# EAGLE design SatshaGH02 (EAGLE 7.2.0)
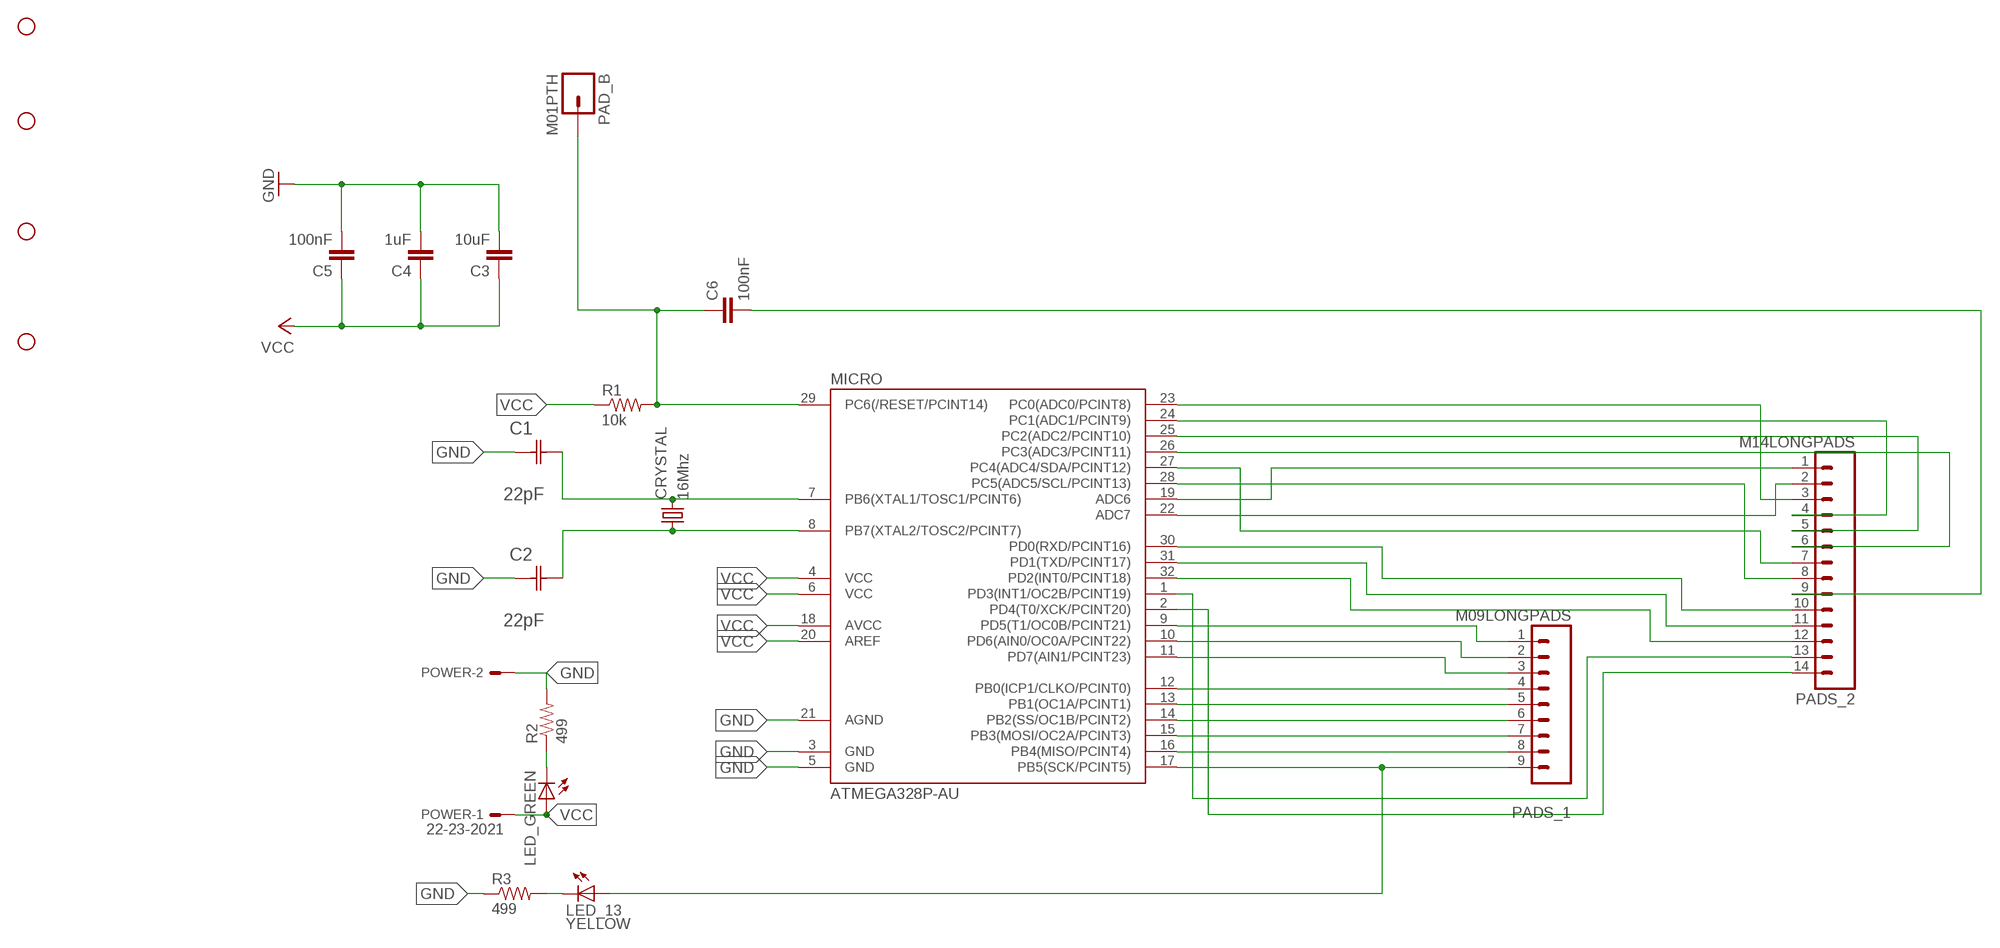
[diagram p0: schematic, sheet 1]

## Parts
C1  22pF  0612ZC225MAT2A  [CAPC3216X178N]
C2  22pF  0612ZC225MAT2A  [CAPC3216X178N]
C3  10uF  CAP1206  [1206]
C4  1uF  CAP1206  [1206]
C5  100nF  CAP1206  [1206]
C6  100nF  CAP1206  [1206]
CRYSTAL  16Mhz  CSM-7X-DU  [CSM-7X-DU]
LED_13  YELLOW  LED1206  [1206]
LED_GREEN  LED1206  [1206]
MICRO  ATMEGA328P-AU  ATMEGA48/88/168-AU  [TQFP32-08]
PAD_B  M01PTH  [1X01]
PADS_1  M09LONGPADS  [1X09_LONGPADS]
PADS_2  M14LONGPADS  [1X14-LONGPADS]
POWER  22-23-2021  [22-23-2021]
R1  10k  RESISTOR1206  [1206]
R2  499  RESISTOR1206  [1206]
R3  499  RESISTOR1206  [1206]
U$1  STAND-OFF  [STAND-OFF]
U$2  STAND-OFF  [STAND-OFF]
U$3  STAND-OFF  [STAND-OFF]
U$4  STAND-OFF  [STAND-OFF]

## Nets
GND: C1.1(C1) C2.1(C1) C3.2 C4.2 C5.2 MICRO.3(GND) MICRO.5(GND) MICRO.21(AGND) POWER.2 R2.2 R3.1
N$1: MICRO.9(PD5(T1/OC0B/PCINT21)) PADS_1.1
N$2: C1.2(C2) CRYSTAL.2 MICRO.7(PB6(XTAL1/TOSC1/PCINT6))
N$3: C6.2 PADS_2.9
N$4: MICRO.10(PD6(AIN0/OC0A/PCINT22)) PADS_1.2
N$5: MICRO.11(PD7(AIN1/PCINT23)) PADS_1.3
N$6: MICRO.12(PB0(ICP1/CLKO/PCINT0)) PADS_1.4
N$7: MICRO.13(PB1(OC1A/PCINT1)) PADS_1.5
N$8: MICRO.14(PB2(SS/OC1B/PCINT2)) PADS_1.6
N$9: C2.2(C2) CRYSTAL.1 MICRO.8(PB7(XTAL2/TOSC2/PCINT7))
N$10: MICRO.15(PB3(MOSI/OC2A/PCINT3)) PADS_1.7
N$11: MICRO.16(PB4(MISO/PCINT4)) PADS_1.8
N$12: LED_13.1(A) MICRO.17(PB5(SCK/PCINT5)) PADS_1.9
N$13: MICRO.19(ADC6) PADS_2.1
N$14: MICRO.22(ADC7) PADS_2.2
N$15: MICRO.23(PC0(ADC0/PCINT8)) PADS_2.3
N$16: MICRO.24(PC1(ADC1/PCINT9)) PADS_2.4
N$17: MICRO.25(PC2(ADC2/PCINT10)) PADS_2.5
N$18: MICRO.26(PC3(ADC3/PCINT11)) PADS_2.6
N$19: MICRO.27(PC4(ADC4/SDA/PCINT12)) PADS_2.7
N$20: MICRO.30(PD0(RXD/PCINT16)) PADS_2.10
N$21: MICRO.31(PD1(TXD/PCINT17)) PADS_2.11
N$22: MICRO.32(PD2(INT0/PCINT18)) PADS_2.12
N$23: MICRO.1(PD3(INT1/OC2B/PCINT19)) PADS_2.13
N$24: MICRO.2(PD4(T0/XCK/PCINT20)) PADS_2.14
N$25: MICRO.28(PC5(ADC5/SCL/PCINT13)) PADS_2.8
N$26: LED_GREEN.2(C) R2.1
N$27: LED_13.2(C) R3.2
N$28: C6.1 MICRO.29(PC6(/RESET/PCINT14)) PAD_B.1 R1.2
VCC: C3.1 C4.1 C5.1 LED_GREEN.1(A) MICRO.4(VCC) MICRO.6(VCC) MICRO.18(AVCC) MICRO.20(AREF) POWER.1 R1.1

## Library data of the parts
C1 C2 = AVX_By_element14_Batch_1:0612ZC225MAT2A: Capacitor 1206; MPN: 0612ZC225MAT2A; OC_FARNELL: -; OC_NEWARK: 12N3209; SUPPLIER: AVX; TOLERANCE: ±20%; VALUE: 2.2µF; VOLTAGERATING: 10V
C3-C6 = 01_SparkFun:CAP: Capacitor
CRYSTAL = 01_FAB_Hello:CSM-7X-DU: SMD CRYSTAL; OC_FARNELL: unknown; OC_NEWARK: unknown
LED_13 LED_GREEN = 01_FAB_Hello:LED
MICRO = atmega8:ATMEGA48/88/168
PAD_B = 01_SparkFun:M01: Header 1
PADS_1 = 01_SparkFun:M09: Header 9 Standard 9-pin 0.1" header. Use with straight break away headers (SKU : PRT-00116), right angle break away headers (PRT-00553), swiss pins (PRT-00743), machine pins (PRT-00117), and female headers (PRT-00115).
PADS_2 = 01_SparkFun:M14: Header 14 Standard 14-pin 0.1" header. Use with straight break away headers (SKU : PRT-00116), right angle break away headers (PRT-00553), swiss pins (PRT-00743), machine pins (PRT-00117), and female headers (PRT-00115).
POWER = con-molex:22-23-2021: .100" (2.54mm) Center Header - 2 Pin; MF: MOLEX; MPN: 22-23-2021; OC_FARNELL: 1462926; OC_NEWARK: 25C3832
R1-R3 = 01_SparkFun:RESISTOR: Resistor
U$1-U$4 = SparkFun:STAND-OFF: Stand Off

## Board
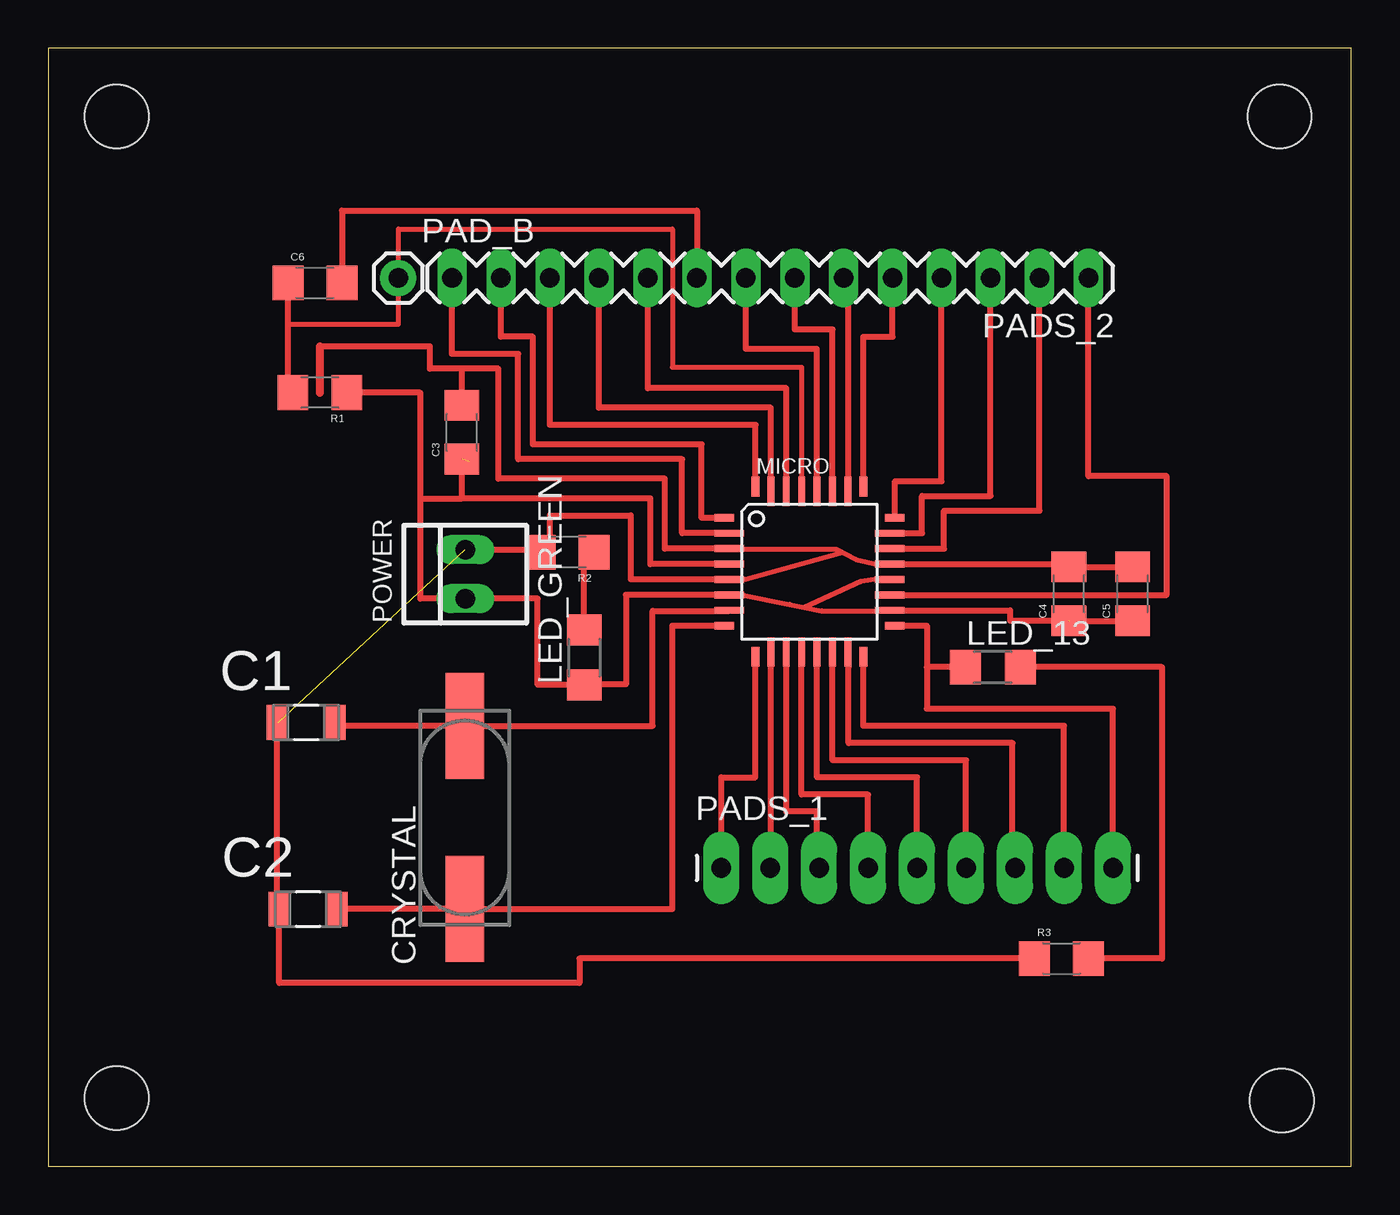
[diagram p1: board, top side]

Size 67.62 x 58.03 mm. Coordinates in mm from the lower left corner, seen from the top.
Outline: 0,0 67.62,0 67.62,58.03 0,58.03 0,0
Copper layers (1*16): Top 0.035mm / dielectric 1.5mm / Bottom 0.035mm
Design rules "default": minimum track width 10mil, minimum drill 24mil, track to track 8mil, track to pad 8mil, pad to pad 8mil, via to via 8mil, smd to smd 8mil, copper to edge 40mil, drill to drill 8mil, minimum pad ring 10mil, minimum via ring 8mil, stop-mask expansion 4mil, vias tented up to drill 0mil, thermal gap 10mil

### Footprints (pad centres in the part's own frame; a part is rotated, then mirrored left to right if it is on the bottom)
CAPC3216X178N = smd 1.118 x 1.803: 1 -1.499,0; 2 1.499,0
1206 = smd 1.6 x 1.8: 1 -1.4,0; 2 1.4,0
CSM-7X-DU = smd 5.5 x 2: 1 -4.75,0; 2 4.75,0
1206' = smd 1.6 x 1.803: 1 -1.422,0; 2 1.422,0
TQFP32-08 = smd 1.016 x 0.406: 1 -4.42,2.8; 8 -4.42,-2.8; 17 4.42,-2.8; 24 4.42,2.8 | smd 1.524 x 0.356: 2 -4.166,2; 3 -4.166,1.2; 4 -4.166,0.4; 5 -4.166,-0.4; 6 -4.166,-1.2; 7 -4.166,-2; 18 4.166,-2; 19 4.166,-1.2; 20 4.166,-0.4; 21 4.166,0.4; 22 4.166,1.2; 23 4.166,2 | smd 0.406 x 1.016: 9 -2.8,-4.42; 16 2.8,-4.42; 25 2.8,4.42; 32 -2.8,4.42 | smd 0.356 x 1.524: 10 -2,-4.166; 11 -1.2,-4.166; 12 -0.4,-4.166; 13 0.4,-4.166; 14 1.2,-4.166; 15 2,-4.166; 26 2,4.166; 27 1.2,4.166; 28 0.4,4.166; 29 -0.4,4.166; 30 -1.2,4.166; 31 -2,4.166
1X01 = drill 1.016 pad 1.88: 1 0,0
1X09_LONGPADS = drill 1.016 pad 1.88 long: 1 0,0; 2 2.54,0; 3 5.08,0; 4 7.62,0; 5 10.16,0; 6 12.7,0; 7 15.24,0; 8 17.78,0; 9 20.32,0
1X14-LONGPADS = drill 1.016 long: 1 0,0; 2 2.54,0; 3 5.08,0; 4 7.62,0; 5 10.16,0; 6 12.7,0; 7 15.24,0; 8 17.78,0; 9 20.32,0; 10 22.86,0; 11 25.4,0; 12 27.94,0; 13 30.48,0; 14 33.02,0
22-23-2021 = drill 1 long: 1 -1.27,0; 2 1.27,0
STAND-OFF = hole 3.302: 0,0

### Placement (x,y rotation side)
C1  13.39,23.04 0 top
C2  13.49,13.36 0 top
C3  21.46,38.1 90 top
C4  52.96,29.72 90 top
C5  56.26,29.72 90 top
C6  13.84,45.85 0 top
CRYSTAL  21.62,18.11 90 top
LED_13  YELLOW  [1206']  49.02,25.91 0 top
LED_GREEN  [1206']  27.81,26.42 90 top
MICRO  39.5,30.86 0 top
PAD_B  18.16,46.1 0 top
PADS_1  34.92,15.49 0 top
PADS_2  53.98,46.1 180 top
POWER  21.64,30.73 90 top
R1  14.1,40.16 180 top
R2  26.92,31.88 180 top
R3  52.58,10.79 0 top
U$1  3.56,3.56 0 top
U$2  3.56,54.48 0 top
U$3  63.88,54.48 0 top
U$4  64.01,3.43 0 top

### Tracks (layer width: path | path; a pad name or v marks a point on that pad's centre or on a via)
GND  (1 unrouted)
  Top 0.254: MICRO.3 35.36,32.03 40.88,32.03 | 40.88,32.03 41.91,31.5 43.05,31.24 | 35.94,30.48 36.2,30.48 41.07,31.83 | 41.07,31.83 41.21,31.86 | 40.88,32.03 41.07,31.83
  Top 0.305: MICRO.5 | MICRO.21 | C1.1 11.89,13.36 C2.1 11.99,9.53 27.56,9.53 27.56,10.79 R3.1 | C1.1 11.81,23.04 | MICRO.5 35.33,30.48 30.23,30.48 30.23,33.78 26.03,33.78 26.03,31.75 R2.2 26.03,32 POWER.2 | C1.1 11.94,23.04 | MICRO.21 52.96,31.26 C4.2 C5.2 | 35.94,30.48 MICRO.5 | MICRO.21 43.05,31.24 | MICRO.3 32,32.06 32,35.69 23.37,35.69 23.37,41.4 21.46,41.4 | 21.46,41.4 19.81,41.4 19.81,42.55 14.1,42.55 | C3.2 21.46,41.4
  Top 0.406: 14.1,42.55 14.1,40.13
N$1
  Top 0.305: PADS_1.1 34.92,20.19 36.7,20.19 MICRO.9
N$2
  Top 0.305: 14.88,22.86 C1.2 14.88,22.86 | MICRO.7 35.33,28.83 31.37,28.83 31.37,22.86 CRYSTAL.2 14.88,22.86
N$3
  Top 0.305: PADS_2.9 33.66,49.61 15.24,49.61 C6.2
N$4
  Top 0.305: PADS_1.2 37.5,15.49 MICRO.10
N$5
  Top 0.305: PADS_1.3 39.88,15.49 39.88,18.41 38.3,18.41 MICRO.11
N$6
  Top 0.305: 39.12,26.7 MICRO.12 39.1,19.3 42.54,19.3 PADS_1.4
N$7
  Top 0.305: PADS_1.5 45.09,20.19 39.9,20.19 MICRO.13
N$8
  Top 0.305: PADS_1.6 47.62,21.08 40.7,21.08 MICRO.14
N$9
  Top 0.305: 14.99,13.34 C2.2 | MICRO.8 32.38,28.07 32.38,13.36 CRYSTAL.1 C2.2 | C2.2
N$10
  Top 0.305: PADS_1.7 50.04,15.49 50.04,21.97 41.53,21.97 41.53,25.91 MICRO.15
N$11
  Top 0.305: MICRO.16 42.3,22.86 52.7,22.86 PADS_1.8
N$12
  Top 0.305: PADS_1.9 55.24,23.75 45.59,23.75 45.59,25.91 | LED_13.1 45.59,25.91 | MICRO.17 45.59,28.06 45.59,25.91
N$13
  Top 0.305: MICRO.19 58.04,29.66 58.04,35.81 53.98,35.81 PADS_2.1
N$14
  Top 0.305: MICRO.22 46.48,32.06 46.48,34.04 51.43,34.04 PADS_2.2
N$15
  Top 0.305: MICRO.23 45.34,32.86 45.34,34.8 48.89,34.8 PADS_2.3
N$16
  Top 0.305: PADS_2.4 46.35,35.56 43.94,35.56 43.94,33.66 MICRO.24
N$17
  Top 0.305: MICRO.25 42.29,43.05 43.81,43.05 PADS_2.5
N$18
  Top 0.305: MICRO.26 41.53,35.03 41.53,45.21 arc-90 41.27,45.47 PADS_2.6
N$19
  Top 0.305: MICRO.27 40.7,43.43 38.73,43.43 PADS_2.7
N$20
  Top 0.305: MICRO.30 38.3,40.39 31.11,40.39 PADS_2.10
N$21
  Top 0.305: MICRO.31 37.5,39.37 28.57,39.37 PADS_2.11
N$22
  Top 0.305: PADS_2.12 26.03,38.48 36.7,38.48 MICRO.32
N$23
  Top 0.305: MICRO.1 33.91,33.66 33.91,37.47 25.15,37.47 25.15,43.05 23.49,43.05 PADS_2.13
N$24
  Top 0.305: MICRO.2 32.89,32.86 32.89,36.7 24.38,36.7 24.38,42.16 20.95,42.16 PADS_2.14
N$25
  Top 0.305: MICRO.28 39.88,35.03 39.88,42.42 36.2,42.42 PADS_2.8
N$26
  Top 0.305: 28.7,31.62 R2.1 28.32,31.5 27.81,31.5 LED_GREEN.2
N$27
  Top 0.305: R3.2 57.79,10.79 57.79,25.91 LED_13.2
N$28
  Top 0.254: MICRO.29 39.1,41.48 32.38,41.48 32.38,48.64 18.16,48.64 PAD_B.1 18.16,43.69 12.44,43.69
  Top 0.305: R1.2 12.44,40.16 12.44,43.69 C6.1
VCC  (2 unrouted)
  Top 0.254: 36.02,29.67 38.47,29.17 39.23,29.01 | 39.23,29.01 40.13,28.83 43.66,28.83 | MICRO.20 43.05,30.46 43.05,30.48 42.16,30.35 39.23,29.01
  Top 0.305: MICRO.18 | MICRO.20 43.05,30.48 | MICRO.4 31.24,31.26 31.24,34.67 21.46,34.67 | 19.3,34.67 19.3,40.16 R1.1 | 19.3,34.67 19.3,29.46 POWER.1 25.4,29.46 25.4,24.99 LED_GREEN.1 27.81,25.02 29.97,25.02 29.97,29.66 MICRO.6 36.02,29.67 | 43.66,28.83 MICRO.18 | MICRO.18 49.91,28.86 49.91,28.32 C4.1 | 21.84,36.57 21.84,36.45 | 19.3,34.67 21.46,34.67 | 21.46,34.67 C3.1 | C4.1 C5.1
